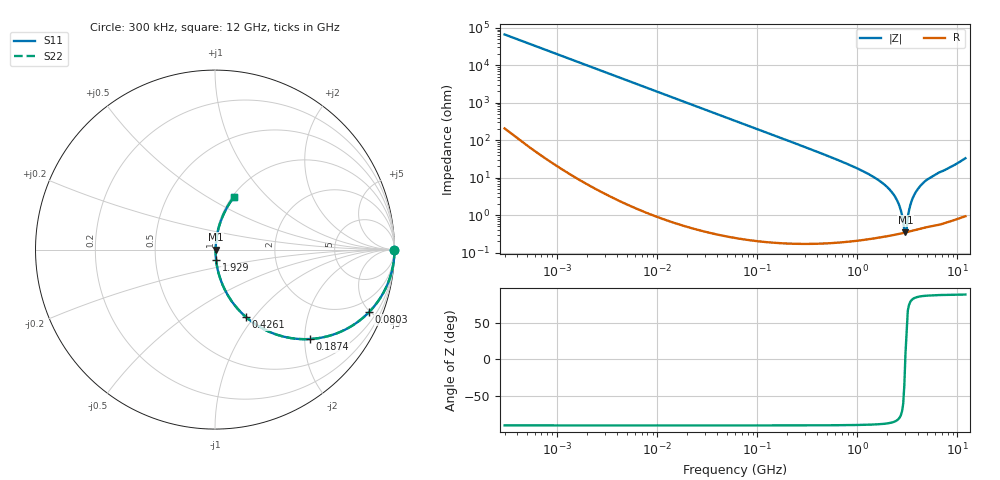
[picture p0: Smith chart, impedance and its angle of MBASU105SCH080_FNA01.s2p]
! MBASU105SCH080_FNA01  S-PARAMETER MODEL  ( Standard Model )
! Model Generated by TAIYO YUDEN Corporation (http://www.ty-top.com)
! Version 1.0
! TAIYO YUDEN Control No. 230609
! Copyright(c) 2023 TAIYO YUDEN CO.,LTD. All Rights Reserved.
! Product Description (link to TY-COMPAS)
! https://ds.yuden.co.jp/TYCOMPAS/or/detail?pn=MBASU105SCH080CFNA01&u=M
! Products Name : Multilayer Ceramic Capacitors
! Characteristics :
!  Capacitance : 8 [pF] , Rated Voltage : 50 [V] , TCC : CH / C0H
!  Case Size : 1.0 x 0.5 / 0.039 x 0.02 [mm/inch] , Thickness : 0.5 / 0.02 [mm/inch]
!  (Conditions: Temperature = 25 [degC] , DC Bias Voltage = 0 [V])
! External Node Assignments :
!  1  o---| |---o  2
! GND o---------o GND
! Frequency Range : 0.3MHz  -  12000MHz  [ 401 STEP ]
# MHZ S RI R 50
! Freq[MHz].  S11 Real  S11 Imag  S21 Real  S21 Imag  S12 Real  S12 Imag  S22 Real  S22 Imag
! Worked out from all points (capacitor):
!   401 points, 300 kHz to 12 GHz, reference 50 ohm
!   read as one part in series: C = 8 pF near 316.3 kHz
!   lowest |Z| = 351 mohm at 3.026 GHz (marker M1)
!   series resonance near 3.013 GHz, so ESL is about 350 pH
!   S11 on the Smith chart (normalised r, x): 300 kHz: open; 80.3 MHz: 1.00, -4.95; 187.4 MHz: 1.00, -2.11; 426.1 MHz: 1.00, -0.91; 1.929 GHz: 1.01, -0.12; 12 GHz: 1.02, +0.66
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0.3  1 -0.00151  6.97e-06 0.00151  6.97e-06 0.00151  1 -0.00151
1.769972  0.9999 -0.0089  8.55e-05 0.0089  8.55e-05 0.0089  0.9999 -0.0089
10.44266  0.9972 -0.0523  0.00277 0.0523  0.00277 0.0523  0.9972 -0.0523
27.10171  0.9817 -0.1337  0.0183 0.1337  0.0183 0.1337  0.9817 -0.1337
60  0.9164 -0.2764  0.0836 0.2764  0.0836 0.2764  0.9164 -0.2764
80.29859  0.8595 -0.347  0.1405 0.347  0.1405 0.347  0.8595 -0.347
187.4445  0.5277 -0.4984  0.4723 0.4984  0.4723 0.4984  0.5277 -0.4984
353.9943  0.2357 -0.4229  0.7643 0.4229  0.7643 0.4229  0.2357 -0.4229
426.1204  0.174 -0.3772  0.826 0.3772  0.826 0.3772  0.174 -0.3772
1105.905  0.0256 -0.1512  0.9744 0.1512  0.9744 0.1512  0.0256 -0.1512
1928.972  0.00633 -0.06  0.9937 0.06  0.9937 0.06  0.00633 -0.06
2088.533  0.0052 -0.0487  0.9948 0.0487  0.9948 0.0487  0.0052 -0.0487
2514.07  0.00365 -0.0234  0.9964 0.0234  0.9964 0.0234  0.00365 -0.0234
2650.866  0.00346 -0.0164  0.9965 0.0164  0.9965 0.0164  0.00346 -0.0164
2947.191  0.00341 -0.00238  0.9966 0.00238  0.9966 0.00238  0.00341 -0.00238
3026.31  0.00346 0.000502  0.9965 -0.000502  0.9965 -0.000502  0.00346 0.000502
3107.553  0.00352 0.00259  0.9965 -0.00259  0.9965 -0.00259  0.00352 0.00259
3364.605  0.00401 0.0172  0.996 -0.0172  0.996 -0.0172  0.00401 0.0172
3547.679  0.00456 0.0267  0.9954 -0.0267  0.9954 -0.0267  0.00456 0.0267
4270.516  0.00802 0.0603  0.992 -0.0603  0.992 -0.0603  0.00802 0.0603
6026.253  0.0197 0.1188  0.9803 -0.1188  0.9803 -0.1188  0.0197 0.1188
12000  0.1051 0.2928  0.8949 -0.2928  0.8949 -0.2928  0.1051 0.2928
